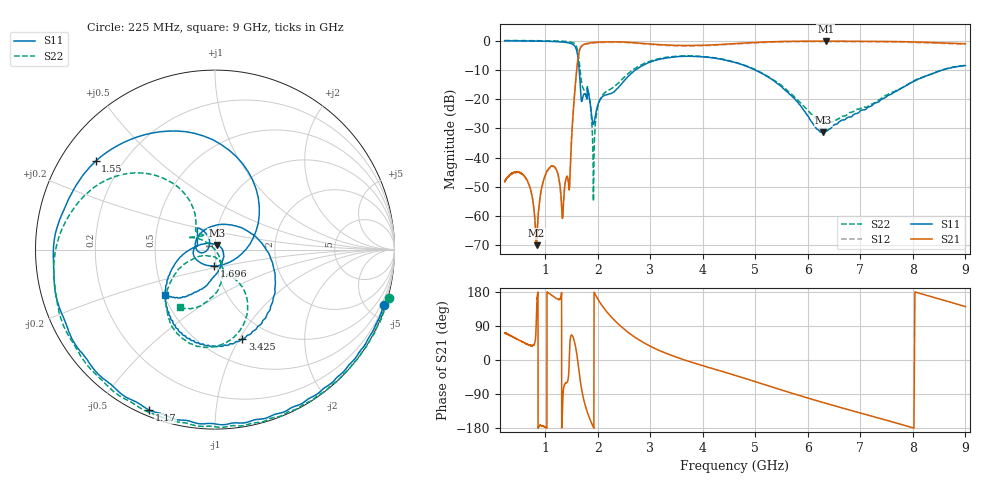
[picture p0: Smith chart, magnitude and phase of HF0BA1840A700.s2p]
!Agilent Technologies,E8358A,US41080443,A.07.50.56
!Agilent E8358A: A.07.50.56
!Date: Monday, May 09, 2016 11:54:42
!Correction: S11(Full 2 Port(1,2))
!S21(Full 2 Port(1,2))
!S12(Full 2 Port(1,2))
!S22(Full 2 Port(1,2))
!S2P File: Measurements: S11, S21, S12, S22:Log Frequency Sweep
# Hz S  dB  R 50
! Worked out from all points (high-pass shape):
!   1601 points, 225 MHz to 9 GHz, reference 50 ohm
!   highest |S21| = -0.20 dB at 6.339 GHz (marker M1); lowest = -70.0 dB at 833.5 MHz (marker M2)
!   |S21| within 3 dB of the highest: 1.653 GHz to end of sweep
!   lowest |S11| = -31.4 dB at 6.296 GHz (marker M3), VSWR 1.06, Z = 50.9 + j2.56 ohm
!   |S11| at or under -10 dB: 1.645 GHz to 2.723 GHz (1.078 GHz wide, 49.4 % of centre); 4.984 GHz to 8.576 GHz (3.592 GHz wide, 53 % of centre)
!   |S22| runs from -54.9 to 0.0 dB; largest |S21 - S12| = 0.021
!   S11 on the Smith chart (normalised r, x): 225 MHz: 0.18, -6.30; 1.17 GHz: 0.03, -0.67; 1.55 GHz: 0.10, +0.33; 1.696 GHz: 0.97, -0.18; 3.425 GHz: 0.76, -1.03; 9 GHz: 0.51, -0.30
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2.25e8  -0.08 -18.0  -48.16 71.7  -48.35 72.0  0.04 -15.5
6.482962e8  -0.13 -53.7  -47.54 41.8  -47.74 42.5  -0.01 -45.7
8.335158e8  -0.19 -71.5  -70.00 126.2  -69.29 129.2  -0.05 -61.0
9.483877e8  -0.25 -84.0  -49.01 -174.4  -49.21 -173.5  -0.09 -71.5
1.169777e9  -0.30 -112.2  -43.05 165.9  -43.23 166.4  -0.10 -95.5
1.330991e9  -0.55 -140.5  -60.44 -113.9  -60.60 -116.4  -0.27 -118.8
1.459576e9  -0.88 -174.4  -50.33 12.9  -50.43 12.8  -0.47 -145.8
1.549745e9  -1.65 143.5  -19.93 51.0  -20.09 51.2  -0.96 -177.2
1.687749e9  -20.64 -68.6  -1.89 -74.0  -2.05 -74.0  -14.00 122.5
1.695549e9  -20.79 -93.8  -1.74 -80.2  -1.91 -80.1  -14.84 125.8
1.833809e9  -18.98 120.0  -0.87 -150.6  -1.04 -150.5  -18.90 147.3
1.920348e9  -28.60 165.7  -0.63 -178.6  -0.79 -178.6  -48.15 -69.3
2.029602e9  -20.69 -172.4  -0.52 154.1  -0.69 154.3  -20.70 -65.6
2.288114e9  -17.76 99.8  -0.44 108.8  -0.60 108.9  -16.08 -62.9
3.152512e9  -6.46 -54.2  -1.33 26.2  -1.50 26.3  -6.22 -75.8
3.425335e9  -5.69 -73.0  -1.61 10.8  -1.79 10.9  -5.48 -86.8
4.622431e9  -7.54 -129.6  -1.03 -40.8  -1.20 -40.8  -7.44 -129.4
6.081681e9  -28.09 121.6  -0.21 -103.7  -0.37 -103.8  -25.28 -139.7
6.295684e9  -31.42 69.1  -0.21 -112.5  -0.38 -112.5  -27.95 -110.2
6.33938e9  -30.97 55.1  -0.20 -114.1  -0.37 -114.2  -28.23 -104.6
7.553438e9  -18.59 -79.4  -0.32 -161.3  -0.48 -161.4  -18.07 -68.8
9e9  -8.54 -137.6  -1.08 140.9  -1.24 140.8  -8.50 -121.2
